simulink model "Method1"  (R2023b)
settings: Solver=FixedStepDiscrete  StartTime=0.0  StopTime=0.5  RelTol=1e-3
undefined symbols (not defined in the file): Datasheet, derived, set
libraries: fl_lib x14, nesl_utility x9, ee_lib x4, slpidlib x1, simulink x1, simulink_extras x1, spspowerguiLib x1

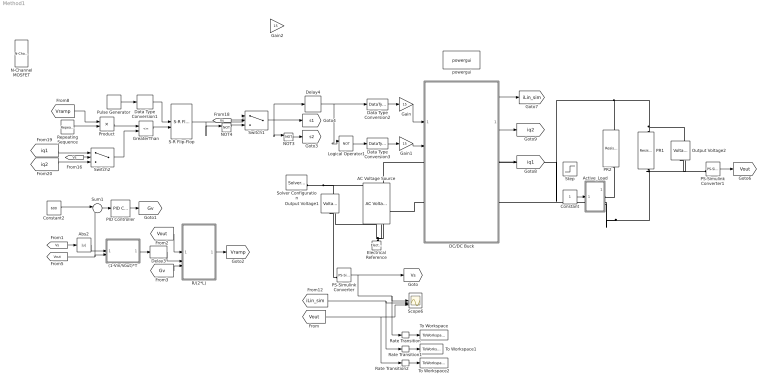
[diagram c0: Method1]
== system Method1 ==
  (1-Vin/Vout)*T : MATLAB Function  TreatAsAtomicUnit=on
  AC Voltage Source : fl_lib/Electrical/Electrical Sources/AC Voltage Source  amp=340 V  shift=0 deg  frequency=50 Hz  omega=0 rad/s
  Abs2 : Abs
  Active_Load : Subsystem
  Constant : Constant
  Constant2 : Constant  Value=600
  DC/DC Buck : Subsystem
  Data Type Conversion1 : DataTypeConversion
  Data Type Conversion2 : DataTypeConversion  OutDataTypeStr=double  RndMeth=Simplest
  Data Type Conversion3 : DataTypeConversion  OutDataTypeStr=double  RndMeth=Simplest
  Delay3 : Delay  DelayLength=10
  Delay4 : Delay  DelayLength=1
  Electrical Reference : fl_lib/Electrical/Electrical Elements/Electrical Reference
  Gain : Gain  Gain=15
  Gain1 : Gain  Gain=15
  Gain2 : Gain  Gain=15
  GreaterThan : RelationalOperator  Operator=<=  OutDataTypeStr=boolean  RndMeth=Simplest
  Logical Operator1 : Logic  Operator=NOT  AllPortsSameDT=off  OutDataTypeStr=boolean
  N-Channel MOSFET : ee_lib/Semiconductors & Converters/N-Channel MOSFET  paramTerminal=ee.enum.mosfet.numberOfTerminals.three  parameterization=ee.enum.mosfet.parameterization.datasheet  Beta=5.0 A/V^2  Rds=0.025 Ohm  Id=6.0 A  Vgs=10 V  Vth=1.7 V  Vth0=1.7 V  lam=0 1/V  gamma_vth=0.5 V^(1/2)  phib=0.5 V  Vth1=1.9071 V  Vbs1=-1 V  Vth2=2.066 V  Vbs2=-2 V  Tmeas=25 degC  Vgs_vec=[-1 0 0.74 1.41 2.02 2.57 3.06 3.51 3.91 4.27 4.6 4.9 5.17 5.41 5.63 5.82 6 6.16 6.31 6.44 6.56 6.67 6.81 6.97 7.16 7.37 7.61 7.89 8.21 8.57 8.98 9.45 9.99 10.61 11.31 12.11 13.03 14.08 15.28 16.65 18.21 20] V  Vds_vec=[0 0.1 1.1 2.1 3.1 4.1 5.1 6.1 7.1 8.1 9.1 10.1 11.1 12.1 13.1 14.1 15.1 16.1 17.1 18.1 19.1 20.1 30 40 50 60 70 80 90 100 110 120 130 140 150 160 170 180 190 200 210 220 230 240 250 260 270 280 290 300 310 320 330 340 350 360 370 380 390 400 410 420 430 440 450 460 470 480 490 500 510 520 530 540 550 560 570 580 590 600 610 620 630 640 650 660 670 680 690 700 710 720 730 740 750 760 770 780 790 8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  Vbs_vec=[0, -4, -6, -12] V  T_vec=[25;100;175] degC  Vth_vec=[.4, 1.2, 1.4, 1.45] V  Vth_mat=[.4, .35; 1.2, 1.15; 1.4, 1.35; 1.45, 1.4] V  Ids_mat=[0, 0, 0, 0, 0, 0, 0; 0, 0, 0, 0, 0, 0, 0; 0, .003, .0038, .0043, .0046, .0048, .0049; 0, .0055, .008, .009, .0095, .01, .0101; 0, .0115, .016, .018, .019, .0195, .02; 0, .0152, .0225, .0265, .028, .0295, .03] A  Ids_mat0=[0, 0, 0, 0, 0, 0, 0; 0, 0, 0, 0, 0, 0, 0; 0, .003, .0038, .0043, .0046, .0048, .0049; 0, .0055, .008, .009, .0095, .01, .0101; 0, .0115, .016, .018, .019, .0195, .02; 0, .0152, .0225, .0265, .028, .0295, .03] A  Ids_mat_3D=zeros(6, 7, 2) A  Ids_mat_3D0=zeros(6, 7, 2) A  IV_table_symmetry=ee.enum.mosfet.symmetricNIV.no  RS=0.0001 Ohm  RD=0.01 Ohm  RB=0.001 Ohm  C_param=ee.enum.mosfet.capacitanceParam.fixedciss  C_GS=270 pF  C_GD=80 pF  C_GB=0 pF  C_DS=0 pF  C_iss=350 pF  C_rss=80 pF  C_oss=0 pF  C_iss_vec=[720, 700, 590, 470, 390, 310] pF  C_rss_vec=[450, 400, 300, 190, 95, 55] pF  C_oss_vec=[900, 810, 690, 420, 270, 170] pF  C_GS_vec=[1.74124643236267e-09 1.74139785874173e-09 1.74141682364474e-09 1.74142233040577e-09 1.74142493418064e-09 1.7414278626316e-09 1.7414275761527e-09 1.7414298043219e-09 1.74143175237841e-09 1.74143352854757e-09 1.74143504370263e-09 1.74144584714017e-09 1.74145200961956e-09 1.74145583570439e-09 1.74145846494405e-09 1.74146041300056e-09 1.74146200454999e-09 1.7414633605501e-09 1.74146455102908e-09 1.74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  C_GD_vec=[9.31507143886424e-11 4.3042397570381e-11 3.61826985653635e-11 3.39318338671921e-11 3.26894767476145e-11 3.1388989876622e-11 3.01595816032143e-11 2.91496479963304e-11 2.82910007121519e-11 2.7539031803229e-11 2.68653098305279e-11 2.22551195235667e-11 1.9597372030282e-11 1.79177717186469e-11 1.67648978742733e-11 1.59040860828687e-11 1.52125260241458e-11 1.46254161714752e-11 1.41080543810653e-11 1.36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  C_GB_vec=[270, 300, 290, 280, 295, 255] pF  C_Vgs_vec=[-5 -3 -1 0 1 3 5 7 9 11 13 15 17 19] V  C_DS_vec=[1.23906948774915e-09;1.10548736992733e-09;1.00848198647898e-09;9.38035425004145e-10;8.74432653406217e-10;8.23194374689189e-10;5.9673868216423e-10;5.57776769053014e-10;5.31439700844806e-10;5.09747372298605e-10;4.9147030511283e-10;3.79228057666435e-10;3.19359971399718e-10;2.80602979827029e-10;2.54110264450675e-10;2.35046564409371e-10;2.20564585038808e-10;2.08974189970118e-10;1.9926781382197e-10;1.9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  C_Vds_vec=[0 1 2 3 4 5 6 7 8 9 10 20 30 40 50 60 70 80 90 100] V  V_GS_for_cap_data=0 V  charge_linearity_param=ee.enum.mosfet.cgdLinearity.constant  C_OX=200 pF  V_C_OX=-0.5 V  charge_linearity_param_vgb=ee.enum.mosfet.cgbLinearity.instantly  charge_linearity_param_with_vgb=ee.enum.mosfet.cgbLinearityWithSeparateCgb.instantly  Di_param=ee.enum.mosfet.diodeParam.no  IsDiode=1e-12 A  Vbi=0.6 V  n=1  Cj0Diode=0 pF  TT=50e-9 s  Tmeas_dio=25 degC  TableTypeNoT=ee.enum.mosfet.tableType.IfMat  TableType=ee.enum.diode.tableType.IfMat  IfVec=[.07, .12, .19, 1.75, 4.24, 7.32, 11.2] A  IfMat="[0 7.5e-06 0.1248618568 0.2497162136 0.3745705704 5.1758758156 13.872619052 25.668336366 40.124473959 56.940499125 75.890523695 96.795450744 119.50820242 143.90493397 169.87938371 197.33902678 226.20234059 256.39679287 287.85731962 320.52514703 354.34686179 389.27366528 425.26076668 462.26688303 500.25382274 539.18613541 579.03081476 619.75704463 661.33598032 703.74055915 746.94533536 790.9263354 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"  VfVecV=[.9, 1.15, 1.25, 1.5, 1.75, 2.17, 2.6, 2.85] V  VfMatV=[.9, 1.15, 1.25, 1.5, 1.75, 2.17, 2.6, 2.85; .58, .68, .75, 1.1, 1.38, 1.77, 2.27, 2.7] V  TjVec=[25 100 175] degC  VfVec=[0 0.75 1.5 2.25 3 3.75 4.5 5.25 6 6.75 7.5 8.25 9 9.75 10.5 11.25 12 12.75 13.5 14.25 15 15.75 16.5 17.25 18 18.75 19.5 20.25 21 21.75 22.5 23.25 24 24.75 25.5 26.25 27 27.75 28.5 29.25 30] V  IfVecV=[.1, .2, .5, 1, 2, 4, 7, 10] A  prmDatasheet=ee.enum.temperatureParameterization.none  prmEquCoeff=ee.enum.temperatureParameterization.none  dVth_dT=-6 mV/K  dVth0_dT=-6 mV/K  Rds_T2=0.037 Ohm  BEXDatasheet=-1.5  BEXEquCoeff=-1.5  etaisDatasheet=3  etaisEquCoeff=3  Tmeas2=125 degC  etaisTabulated=3  TdeviceDatasheet=25 degC  TdeviceEquCoeff=25 degC  TdeviceTabulated=25 degC  enable_faults=simscape.enum.onoff.off  fault_trigger=ee.enum.faults.faultTrigger.temporal  t_fault=inf s  max_permissible_Vgs=inf V  max_permissible_Vds=inf V  max_permissible_Vdb=inf V  max_permissible_Ids=inf A  t_fail_on_Ids=1 s  max_permissible_Idiode=inf A  t_fail_on_Idiode=1 s  max_permissible_dVdt=inf V/s  tau_fault=1e-3 s  fault_types=ee.enum.mosfet.faults.open  fault_types_4T=ee.enum.mosfet.faultsFourTerminals.open  RG_open=1e6 Ohm  RD_open=1000 Ohm  RS_open=1000 Ohm  RB_open=1000 Ohm  GDS_short=1000 1/Ohm  GDB_short=1000 1/Ohm  GSB_short=1000 1/Ohm  location_GOS=0  G_GOS=1000 1/Ohm  D_GOS=ee.enum.include.no  Is_GOS=0 A  Vbi_GOS=0.6 V  n_GOS=1  Cj0_GOS=0 pF  TT_GOS=50e-9 s  Beta_scale=100  dVth_faulted=0 V  lam_faulted=0 1/V  gamma_scale=100  dPhib_faulted=0 V  Vgs_vec_faulted=[-1, -.5, 2, 3, 4, 5] V  Vds_vec_faulted=[0, 2, 4, 8, 12, 16, 20] V  Vbs_vec_faulted=[0, -4, -6, -12] V  Vth_vec_faulted=[.4, 1.2, 1.4, 1.45] V  Vth_mat_faulted=[.4, .35; 1.2, 1.15; 1.4, 1.35; 1.45, 1.4] V  Ids_mat_faulted=[0, 0, 0, 0, 0, 0, 0; 0, 0, 0, 0, 0, 0, 0; 0, .003, .0038, .0043, .0046, .0048, .0049; 0, .0055, .008, .009, .0095, .01, .0101; 0, .0115, .016, .018, .019, .0195, .02; 0, .0152, .0225, .0265, .028, .0295, .03] A  Ids_mat0_faulted=[0, 0, 0, 0, 0, 0, 0; 0, 0, 0, 0, 0, 0, 0; 0, .003, .0038, .0043, .0046, .0048, .0049; 0, .0055, .008, .009, .0095, .01, .0101; 0, .0115, .016, .018, .019, .0195, .02; 0, .0152, .0225, .0265, .028, .0295, .03] A  Ids_mat_3D_faulted=zeros(6, 7, 2) A  Ids_mat_3D0_faulted=zeros(6, 7, 2) A  RS_faulted=0.0001 Ohm  RD_faulted=0.01 Ohm  RB_faulted=0.001 Ohm  IsDiode_faulted=0 A  Vbi_faulted=0.6 V  n_faulted=1  Cj0Diode_scale=100  TT_faulted=50e-9 s  IfVec_faulted=[.07, .12, .19, 1.75, 4.24, 7.32, 11.2] A  IfMat_faulted=[.07, .12, .19, 1.75, 4.24, 7.32, 11.2; .16, .3, .72, 2.14, 4.02, 6.35, 9.12] A  VfVecV_faulted=[.9, 1.15, 1.25, 1.5, 1.75, 2.17, 2.6, 2.85] V  VfMatV_faulted=[.9, 1.15, 1.25, 1.5, 1.75, 2.17, 2.6, 2.85; .58, .68, .75, 1.1, 1.38, 1.77, 2.27, 2.7] V  VfVec_faulted=[.5, .7, .9, 1.3, 1.7, 2.1, 2.5] V  IfVecV_faulted=[.1, .2, .5, 1, 2, 4, 7, 10] A  C_GS_scale=100  C_GD_scale=100  C_GB_scale=100  C_DS_scale=100  C_OX_scale=100  V_C_OX_faulted=-0.5 V  C_iss_vec_faulted=[720, 700, 590, 470, 390, 310] pF  C_rss_vec_faulted=[450, 400, 300, 190, 95, 55] pF  C_oss_vec_faulted=[900, 810, 690, 420, 270, 170] pF  C_GS_vec_faulted=[270, 300, 290, 280, 295, 255] pF  C_GD_vec_faulted=[450, 400, 300, 190, 95, 55] pF  C_GB_vec_faulted=[270, 300, 290, 280, 295, 255] pF  C_Vgs_vec_faulted=0 V  C_DS_vec_faulted=[450, 410, 390, 230, 175, 115] pF  C_Vds_vec_faulted=[.1, .3, 1, 3, 10, 30] V  V_GS_for_cap_data_faulted=0 V  i_g_specify=off  i_g_priority=None  i_g=0 A  i_g_nominal_specify=off  i_g_nominal_unit=A  i_g_nominal_value=1  i_d_specify=off  i_d_priority=None  i_d=0 A  i_d_nominal_specify=off  i_d_nominal_unit=A  i_d_nominal_value=1  i_b_specify=off  i_b_priority=None  i_b=0 A  i_b_nominal_specify=off  i_b_nominal_unit=A  i_b_nominal_value=1  voltage_gs_specify=off  voltage_gs_priority=None  voltage_gs=0 V  voltage_gs_nominal_specify=off  voltage_gs_nominal_unit=V  voltage_gs_nominal_value=1  voltage_ds_specify=off  voltage_ds_priority=None  voltage_ds=0 V  voltage_ds_nominal_specify=off  voltage_ds_nominal_unit=V  voltage_ds_nominal_value=1  voltage_bs_specify=off  voltage_bs_priority=None  voltage_bs=0 V  voltage_bs_nominal_specify=off  voltage_bs_nominal_unit=V  voltage_bs_nominal_value=1  v_Cgs_specify=off  v_Cgs_priority=High  v_Cgs=0 V  v_Cgs_nominal_specify=off  v_Cgs_nominal_unit=V  v_Cgs_nominal_value=1  v_Cds_specify=off  v_Cds_priority=High  v_Cds=0 V  v_Cds_nominal_specify=off  v_Cds_nominal_unit=V  v_Cds_nominal_value=1  v_Cbs_specify=off  v_Cbs_priority=High  v_Cbs=0 V  v_Cbs_nominal_specify=off  v_Cbs_nominal_unit=V  v_Cbs_nominal_value=1  faulted_specify=off  faulted_priority=None  faulted=0  faulted_nominal_specify=off  faulted_nominal_unit=1  faulted_nominal_value=1  thermal_network_parameterization=ee.enum.thermalNetworkTopology.junctionCase  Rth=[0, 10] K/W  Rth_Cauer=[1, 3, 10] K/W  Rth_Foster=[4, 6] K/W  thermal_mass_parameterization=ee.enum.thermalNetwork.timeconstant  thermal_mass=[0, 1] J/K  thermal_mass_Cauer=[.1, .3, 1] J/K  thermal_mass_Foster=[1.5, 3] J/K  thermal_time_constant=[0, 10] s  thermal_time_constant_Cauer=[1, 3, 10] s  thermal_time_constant_Foster=[6, 18] s  thermal_mass_initial_temperatures=[25, 25] degC  thermal_mass_initial_temperatures_Cauer=[25, 25, 25] degC  Tvec_initial_Foster=[25, 25, 25, 25] degC  max_permissible_temperature=inf K  t_fail_on_temperature=1 s  betaref=18 A/V^2  Vfbref=-1.1 V  gamma=3.5 V^(1/2)  phib2ref=1 V  thesatref=0.4 1/V  alpha=0  Vp=5e-2 V  thesrref=0 1/V  m=8  Tref=25 degC  Rsref=2e-3 Ohm  Rdref=0.17 Ohm  Rgref=8.4 Ohm  Rbref=2e-3 Ohm  Cox=1500 pF  Cgso=100 pF  Cgdo=14 pF  Isref=5.2e-13 A  Cj0=480 pF  Tprm=1  etabet=1.3  Stvfb=5e-4 V/K  Stphib=-8.5e-4 V/K  etasat=1.04  etasr=0.65  etar=0.95  etais=3  Tsim=25 degC  Ig_specify=off  Ig_priority=None  Ig=0 A  Ig_nominal_specify=off  Ig_nominal_unit=A  Ig_nominal_value=1  Ids_specify=off  Ids_priority=None  Ids=0 A  Ids_nominal_specify=off  Ids_nominal_unit=A  Ids_nominal_value=1  Ib_specify=off  Ib_priority=None  Ib=0 A  Ib_nominal_specify=off  Ib_nominal_unit=A  Ib_nominal_value=1  V_gs_specify=off  V_gs_priority=None  V_gs=0 V  V_gs_nominal_specify=off  V_gs_nominal_unit=V  V_gs_nominal_value=1  V_ds_specify=off  V_ds_priority=None  V_ds=0 V  V_ds_nominal_specify=off  V_ds_nominal_unit=V  V_ds_nominal_value=1  V_bs_specify=off  V_bs_priority=None  V_bs=0 V  V_bs_nominal_specify=off  V_bs_nominal_unit=V  V_bs_nominal_value=1  QGoverCox_specify=off  QGoverCox_priority=None  QGoverCox=0 V  QGoverCox_nominal_specify=off  QGoverCox_nominal_unit=V  QGoverCox_nominal_value=1  QDoverCox_specify=off  QDoverCox_priority=None  QDoverCox=0 V  QDoverCox_nominal_specify=off  QDoverCox_nominal_unit=V  QDoverCox_nominal_value=1  QBoverCox_specify=off  QBoverCox_priority=None  QBoverCox=0 V  QBoverCox_nominal_specify=off  QBoverCox_nominal_unit=V  QBoverCox_nominal_value=1  T0=[25, 25] degC  T0_Cauer=[25, 25, 25] degC
  NOT3 : Logic  Operator=NOT  IconShape=distinctive  AllPortsSameDT=off  OutDataTypeStr=boolean
  NOT4 : Logic  Operator=NOT  IconShape=distinctive  AllPortsSameDT=off  OutDataTypeStr=boolean
  Output Voltage1 : fl_lib/Electrical/Electrical Sensors/Voltage Sensor  Priority=0
  Output Voltage2 : fl_lib/Electrical/Electrical Sensors/Voltage Sensor  Priority=0
  PID Controller : slpidlib/PID Controller  Controller=PID  Form=Parallel  TimeDomain=Discrete-time  UseExternalTs=off  SampleTime=-1  IntegratorMethod=Forward Euler  FilterMethod=Forward Euler  ControllerParametersSource=internal  P=0  I=0.01  UseKiTs=off  D=0  N=100  UseFilter=on  TunerSelectOption=Transfer Function Based (PID Tuner App)  InitialConditionSource=internal  InitialConditionForIntegrator=0  InitialConditionForFilter=0  DifferentiatorICPrevScaledInput=0  ExternalReset=none  TrackingMode=off  Kt=1  LimitOutput=off  SatLimitsSource=internal  UpperSaturationLimit=0.9  LowerSaturationLimit=0  LinearizeAsGain=on  AntiWindupMode=none  Kb=1  LimitIntegrator=off  UpperIntegratorSaturationLimit=inf  LowerIntegratorSaturationLimit=-inf  POutMin=[]  POutMax=[]  IOutMin=[]  IOutMax=[]  DOutMin=[]  DOutMax=[]  NOutMin=[]  NOutMax=[]  SumOutMin=[]  SumOutMax=[]  SaturationOutMin=[]  SaturationOutMax=[]  PParamMin=[]  PParamMax=[]  IParamMin=[]  IParamMax=[]  DParamMin=[]  DParamMax=[]  NParamMin=[]  NParamMax=[]  KbParamMin=[]  KbParamMax=[]  KtParamMin=[]  KtParamMax=[]  KbOutMin=[]  KbOutMax=[]  KtOutMin=[]  KtOutMax=[]  IntegratorOutMin=[]  IntegratorOutMax=[]  FilterOutMin=[]  FilterOutMax=[]  SumI1OutMin=[]  SumI1OutMax=[]  SumI2OutMin=[]  SumI2OutMax=[]  SumI3OutMin=[]  SumI3OutMax=[]  SumI4OutMin=[]  SumI4OutMax=[]  SumDOutMin=[]  SumDOutMax=[]  DifferentiatorOutMin=[]  DifferentiatorOutMax=[]  FilterDiffOutCoefMin=[]  FilterDiffOutCoefMax=[]  ReciprocalOutMin=[]  ReciprocalOutMax=[]  SumDenOutMin=[]  SumDenOutMax=[]  SumNumOutMin=[]  SumNumOutMax=[]  DivideOutMin=[]  DivideOutMax=[]  UdiffTsProdOutMin=[]  UdiffTsProdOutMax=[]  NTsProdOutMin=[]  NTsProdOutMax=[]  UintegralTsProdOutMin=[]  UintegralTsProdOutMax=[]  UngainTsProdOutMin=[]  UngainTsProdOutMax=[]  ClampingZeroOutDataTypeStr=Inherit: Inherit via back propagation  ClampingZeroOutMin=[]  ClampingZeroOutMax=[]  FilterDenConstantOutDataTypeStr=Inherit: Inherit via back propagation  FilterDenConstantOutMin=[]  FilterDenConstantOutMax=[]  PCopyOutDataTypeStr=Inherit: Inherit via back propagation  PCopyOutMin=[]  PCopyOutMax=[]  NCopyOutDataTypeStr=Inherit: Inherit via back propagation  NCopyOutMin=[]  NCopyOutMax=[]  IntegratorContinuousStateAttributes=''  IntegratorStateMustResolveToSignalObject=off  IntegratorRTWStateStorageClass=Auto  FilterContinuousStateAttributes=''  FilterStateMustResolveToSignalObject=off  FilterRTWStateStorageClass=Auto  ParallelPVariant=InternalParameters  IdealPVariant=Disabled  IVariant=InternalParameters  DVariant=InternalParameters  IntegratorVariant=Discrete  SatVariant=Disabled  AWVariant=Passthrough  PCopyVariant=Disabled  TRVariant=Disabled  FdbkBlocksVariant=Forward  IdealPFdbkVariant=Disabled  SatFdbkVariant=Disabled  DerivativeFilterVariant=ForwardEulerFilter  NVariant=InternalParameters  NCopyVariant=Disabled  FilterICVariant=InternalICsFilter  IntegratorICVariant=InternalICs  ExternalResetVariant=Disabled  TRSumVariant=Passthrough  SumFdbkVariant=Disabled  SumVariant=Sum_PID  TsampFilterVariant=InternalTs  TsampNgainVariant=Passthrough  TsampIntegralVariant=Disabled_SignalSpec  ExternalSaturationOutDataTypeStr=Inherit: Same as second input
  PR1 : fl_lib/Electrical/Electrical Elements/Resistor  R=360 Ohm  i_specify=off  i_priority=None  i=0 A  i_nominal_specify=off  i_nominal_unit=A  i_nominal_value=1  v_specify=off  v_priority=None  v=0 V  v_nominal_specify=off  v_nominal_unit=V  v_nominal_value=1
  PR2 : fl_lib/Electrical/Electrical Elements/Resistor  R=360 Ohm  i_specify=off  i_priority=None  i=0 A  i_nominal_specify=off  i_nominal_unit=A  i_nominal_value=1  v_specify=off  v_priority=None  v=0 V  v_nominal_specify=off  v_nominal_unit=V  v_nominal_value=1
  PS-Simulink Converter : nesl_utility/PS-Simulink Converter  Priority=2  PhysicalDomain=network_engine_domain  SubClassName=ps_output  LeftPortType=input  RightPortType=output  PseudoPeriodic=off  Frequencies=[]  VectorFormat=1-D array  Unit=1  AffineConversion=off
  PS-Simulink Converter1 : nesl_utility/PS-Simulink Converter  Priority=2  PhysicalDomain=network_engine_domain  SubClassName=ps_output  LeftPortType=input  RightPortType=output  PseudoPeriodic=off  Frequencies=[]  VectorFormat=1-D array  Unit=1  AffineConversion=off
  Product : Product
  Pulse Generator : DiscretePulseGenerator  PulseType=Time based  Period=10e-6
  R/(2*L) : MATLAB Function  TreatAsAtomicUnit=on
  Rate Transition : RateTransition  OutPortSampleTime=1e-5
  Rate Transition1 : RateTransition  OutPortSampleTime=1e-5
  Rate Transition2 : RateTransition  OutPortSampleTime=1e-5
  Repeating Sequence : simulink/Sources/Repeating Sequence  rep_seq_t=[0 10e-6]  rep_seq_y=[1 0]
  S-R Flip-Flop : simulink_extras/Flip Flops/S-R Flip-Flop  initial_condition=0
  Scope6 : Scope  NumInputPorts=3
  Solver Configuration : nesl_utility/Solver Configuration  PhysicalDomain=network_engine_domain  SubClassName=solver  LeftPortType=input  RightPortType=generic  Tones=[]  Harmonics=[]  SimulateNoise=off  Profile=off  UseLocalSampling=off  EnableSwitchedLinearOptims=on  FrequencyDomain=off  UseCCode=off  RelTol=0.001  AbsTol=1e-06  MinStep=1e-09  ToWorkspace=off  RevertToSquareIcSolve=off  NumHomotopyIterations=100  PhasorMode=off  PhasorModeNumHarmonics=1  ConsistencySolver=NEWTON_FTOL  IndexReductionMethod=DerivativeReplacement  DoDC=off  ResidualTolerance=1e-08  ConsistencyTolSource=GLOBAL  ConsistencyAbsTol=0.001  ConsistencyRelTol=0.001  ConsistencyTolFactor=0.001  UseLocalSolver=on  LocalSolverChoice=NE_TRAPEZOIDAL_ADVANCER  ResolveIndetEquations=on  FunctionEvalNumThread=1  LocalSolverSampleTime=1e-7  DoFixedCost=on  MaxNonlinIter=3  MaxModeIter=2  ComputeImpulses=off  ImpulseIterations=2  LinearAlgebra=auto  LinearAlgebraNumThread=0  EquationFormulation=NE_TIME_EF  DelaysMemoryBudget=1024  AutomaticFiltering=on  FilteringTimeConstant=0.001  PartitionStorageMethod=AS_NEEDED  PartitionMemoryBudget=1024  PartitionMethod=ROBUST  MultibodyUseLocalSolver=off  MultibodyLocalSolverChoice=ODE1  MultibodyLocalSolverSampleTime=0.001
  Step : Step  Time=0.2  Before=1  After=0  SampleTime=0
  Sum1 : Sum  Inputs=|+-
  Switch1 : Switch  Criteria=u2 > Threshold
  Switch2 : Switch  Criteria=u2 > Threshold
  To Workspace : ToWorkspace  VariableName=Vs_method1  SaveFormat=Timeseries  SampleTime=-1
  To Workspace1 : ToWorkspace  VariableName=I_method1  SaveFormat=Timeseries  SampleTime=-1
  To Workspace2 : ToWorkspace  VariableName=Vout_method1  SaveFormat=Timeseries  SampleTime=-1
  powergui : spspowerguiLib/powergui  Priority=1  SimulationMode=Continuous  SampleTime=1e-6  frequency=60  Iterations=50  frequencyindice=60  Pbase=100e6  ErrMax=1e-4  UnitsV=kV  UnitsW=MW  buscounter=0  FunctionMessages=off  echomessages=off  EnableUseOfTLC=off  CurrentSourceSwitches=off  DisableSnubberDevices=off  DisableRonSwitches=off  DisableVfSwitches=off  DisplayEquations=off  AutomaticDiscreteSolvers=off  SolverType=Tustin/Backward Euler (TBE)  Interpol=off  ExternalGateDelay=off  methode=off  Ts=100  x0status=blocks  SPID=on  SwTol=0  HookPort=off  NonlinearTolerance=1e-4  nMaxIteration=100  ContinueOnMaxIteration=off  RestoreLinks=warning  ResistiveCurrentMeasurement=off  Frange=[0:2:500]  Ylog=off  Xlog=on  ShowGrid=off  save=off  variable=ZData  structure=0  ZoomFFT=off  StartTime=0.0  cycles=1  DisplayStyle=1  fundamental=60  FreqAxis=off  MaxFrequency=1000  frequencyindicesteady=1  RmsSteady=1  display=off
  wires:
  Logical Operator1/1 -> Data Type Conversion3/1
  Data Type Conversion2/1 -> Gain/1
  Data Type Conversion3/1 -> Gain1/1
  DC/DC Buck/1(I_sensor) -> [iLin_sim]
  Switch1/1 -> Delay4/1, NOT3/1, [s1]
  [Vout] -> Rate Transition2/1, Scope6/3
  [iLin_sim] -> Rate Transition1/1, Scope6/2
  S-R Flip-Flop/1 -> Switch1/1, NOT4/1
  NOT3/1 -> [s2]
  GreaterThan/1 -> S-R Flip-Flop/2
  NOT4/1 -> Switch1/3
  [Vs] -> Switch1/2
  Data Type Conversion1/1 -> S-R Flip-Flop/1
  Pulse Generator/1 -> Data Type Conversion1/1
  Repeating Sequence/1 -> Product/2
  Product/1 -> GreaterThan/1
  PS-Simulink Converter/1 -> [Vs], Rate Transition/1, Scope6/1
  (1-Vin/Vout)*T/1(Ton) -> Delay3/1
  [Gv] -> R/(2*L)/3(Gv)
  Delay3/1 -> R/(2*L)/2(Ton)
  R/(2*L)/1(y) -> [Vramp]
  PID Controller/1 -> [Gv]
  Sum1/1 -> PID Controller/1
  [Vs] -> Abs2/1
  [Vout] -> R/(2*L)/1(Vout)
  Constant2/1 -> Sum1/1
  [Vramp] -> Product/1
  [Vout] -> (1-Vin/Vout)*T/2(Vout), Sum1/2
  PS-Simulink Converter1/1 -> [Vout]
  Abs2/1 -> (1-Vin/Vout)*T/1(Vin)
  [Vs] -> Switch2/2
  [iq2] -> Switch2/3
  [iq1] -> Switch2/1
  Switch2/1 -> GreaterThan/2
  DC/DC Buck/3(iq1) -> [iq1]
  DC/DC Buck/2(iq2) -> [iq2]
  Delay4/1 -> Data Type Conversion2/1, Logical Operator1/1
  Rate Transition/1 -> To Workspace/1
  Rate Transition1/1 -> To Workspace1/1
  Rate Transition2/1 -> To Workspace2/1
  Gain/1 -> DC/DC Buck/1(In1)
  Gain1/1 -> DC/DC Buck/2(In2)
  Constant/1 -> Active_Load/1(In1)
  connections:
  PR1/RConn1 -- Output Voltage2/RConn2 -- Active_Load/RConn2 -- DC/DC Buck/RConn2
  Solver Configuration/RConn1 -- Output Voltage1/LConn1 -- AC Voltage Source/LConn1 -- DC/DC Buck/LConn1
  Electrical Reference/LConn1 -- DC/DC Buck/LConn2 -- Output Voltage1/RConn2 -- AC Voltage Source/RConn1
  PR1/LConn1 -- Output Voltage2/LConn1 -- DC/DC Buck/RConn1 -- PR2/LConn1
  PR2/RConn1 -- Active_Load/RConn1
  PS-Simulink Converter/LConn1 -- Output Voltage1/RConn1
  PS-Simulink Converter1/LConn1 -- Output Voltage2/RConn1

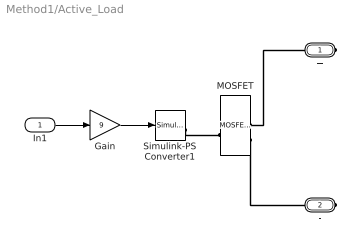
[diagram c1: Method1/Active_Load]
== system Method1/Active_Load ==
  In1 : Inport
  Gain : Gain  Gain=9
  MOSFET : ee_lib/Semiconductors & Converters/MOSFET (Ideal, Switching)  port_option=ee.enum.controlport.ps  Rds=0.2 Ohm  Goff=1e-6 1/Ohm  Vth=3 V  diode_param=ee.enum.converters.protectiondiode.nodynamics  diode_Vf=1.6 V  diode_Ron=0.001 Ohm  diode_Goff=1e-5 1/Ohm  diode_C=5e-8 F  diode_iRM=-235 A  diode_iF=300 A  diode_idot=-100 A/us  diode_trr_param=2  diode_trr_factor=3  diode_trr=70 ns  diode_Qrr=1.5e+3 s*uA  ids_specify=off  ids_priority=None  ids=0 A  ids_nominal_specify=off  ids_nominal_unit=A  ids_nominal_value=1  vds_specify=off  vds_priority=None  vds=0 V  vds_nominal_specify=off  vds_nominal_unit=V  vds_nominal_value=1  vgs_specify=off  vgs_priority=None  vgs=0 V  vgs_nominal_specify=off  vgs_nominal_unit=V  vgs_nominal_value=1  thermal_loss_option=ee.enum.converters.thermalLossOption.constantvalues  Von_data=[0, 1.8, 3.2, 6, 10, 16; 0, 2, 5.5, 9.5, 15, 25] V  Tj=[298.15, 448.15] K  Iout_data=[0, 20, 40, 60, 80, 100] A  Eon_data=[0, 55.04, 124.57, 235.53, 362.12; 0, 71.25, 161.25, 304.88, 468.75] * 1e-6 J  Eoff_data=[0, 18, 30, 56.1, 76.5; 0, 22.5, 37.5, 70.13, 95.63] * 1e-6 J  Eon_data_3D=[zeros(2, 5, 3)] J  Eoff_data_3D=[zeros(2, 5, 3)] J  Tj_loss=[298.15, 448.15] K  Iout_data_loss=[0, 10, 20, 30, 40] A  tabulateWithVds=false  Vds_loss=[0, 150, 300] V  Eon_scalar=22.86e-3 J  Eoff_scalar=17.14e-3 J  Voff=300 V  Iout_scalar=600 A  useCurrentFromPreviousCycle=false  useVoltageFromPreviousCycle=false  diodeModelType=ee.enum.converters.diodeModelType.pwl  diodeTableType=ee.enum.diode.tableType.IfMat  diode_IfMat=[.07, .12, .19, 1.75, 4.24, 7.32, 11.2; .16, .3, .72, 2.14, 4.02, 6.35, 9.12] A  diode_VfMat=[.9, 1.15, 1.25, 1.5, 1.75, 2.17, 2.6, 2.85; .58, .68, .75, 1.1, 1.38, 1.77, 2.27, 2.7] V  diode_TjVec=[25, 125] degC  diode_VfVec=[.5, .7, .9, 1.3, 1.7, 2.1, 2.5] V  diode_IfVec=[.1, .2, .5, 1, 2, 4, 7, 10] A  diode_Vr=-600 V  diode_Ls=150 nH  diode_Erec=0.03 J  diode_rec_loss_model=ee.enum.diode.reverseRecoveryModel.fixed  diode_ErecVal=0 J  diode_scaleWithIandV=true  diode_ErecMat=zeros(2, 3) J  diode_TjrecVec=[298.15, 398.15] K  diode_IfrecVec=[.1, 1, 10] A  diode_IrecVal=10 A  diode_VrecVal=10 V  diode_tFilter=1 / 1000 / 100 s  thermal_network_parameterization=ee.enum.thermalNetworkTopology.external  Rth=[.03, .2] K/W  Rth_Cauer=[.03, .1, .2] K/W  Rth_Foster=[.03, .2] K/W  thermal_mass_parameterization=ee.enum.thermalNetwork.timeconstant  thermal_mass=[3, 25] J/K  thermal_mass_Cauer=[3, 10, 25] J/K  thermal_mass_Foster=[33, 50] J/K  thermal_time_constant=[.1, 5] s  thermal_time_constant_Cauer=[.1, 1, 5] s  thermal_time_constant_Foster=[1, 10] s  thermal_mass_initial_temperatures=[25, 25] degC  thermal_mass_initial_temperatures_Cauer=[25, 25, 25] degC  junction_thermal_mass=0.1 J/K  Tvec_initial_Foster=[25, 25, 25, 25] degC  no_thermal_network=0  junction_temperature_specify=off  junction_temperature_priority=None  junction_temperature=25 degC  junction_temperature_nominal_specify=off  junction_temperature_nominal_unit=degC  junction_temperature_nominal_value=1  Qj_specify=off  Qj_priority=None  Qj=0 W  Qj_nominal_specify=off  Qj_nominal_unit=W  Qj_nominal_value=1  accumulatedSwitchingLosses_specify=off  accumulatedSwitchingLosses_priority=None  accumulatedSwitchingLosses=0 J
  Simulink-PS Converter1 : nesl_utility/Simulink-PS Converter  PhysicalDomain=network_engine_domain  SubClassName=ps_input  LeftPortType=input  RightPortType=output  PseudoPeriodic=off  Frequencies=[]  NoiseDistribution=none  NoiseParameters=[]  Unit=1  AffineConversion=off  FilteringAndDerivatives=provide  SimscapeFilterOrder=1  InputFilterTimeConstant=0.001  UdotUserProvided=0
  + : PMIOPort  Side=Right
  - : PMIOPort  Port=2  Side=Right
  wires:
  In1/1 -> Gain/1
  Gain/1 -> Simulink-PS Converter1/1
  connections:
  MOSFET/RConn2 -- -/RConn1
  MOSFET/RConn1 -- +/RConn1
  Simulink-PS Converter1/RConn1 -- MOSFET/LConn1

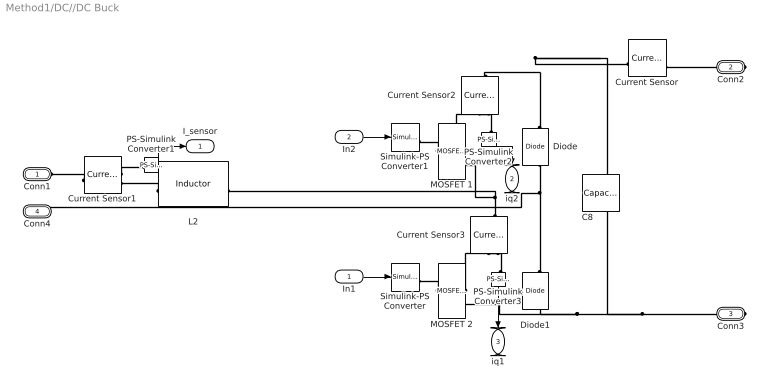
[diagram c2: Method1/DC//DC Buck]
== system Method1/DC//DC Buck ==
  In1 : Inport
  In2 : Inport  Port=2
  C8 : fl_lib/Electrical/Electrical Elements/Capacitor  c=0.1 mF  r=0.15 Ohm  g=0 1/Ohm  i_specify=off  i_priority=None  i=0 A  i_nominal_specify=off  i_nominal_unit=A  i_nominal_value=1  v_specify=off  v_priority=None  v=0 V  v_nominal_specify=off  v_nominal_unit=V  v_nominal_value=1  vc_specify=off  vc_priority=High  vc=0 V  vc_nominal_specify=off  vc_nominal_unit=V  vc_nominal_value=1
  Current Sensor{,1..3} (4 alike) : fl_lib/Electrical/Electrical Sensors/Current Sensor
  Diode : fl_lib/Electrical/Electrical Elements/Diode  Vf=0.6 V  Ron=0.3 Ohm  Goff=1e-8 1/Ohm  i_specify=off  i_priority=None  i=0 A  i_nominal_specify=off  i_nominal_unit=A  i_nominal_value=1  v_specify=off  v_priority=None  v=0 V  v_nominal_specify=off  v_nominal_unit=V  v_nominal_value=1
  Diode1 : fl_lib/Electrical/Electrical Elements/Diode  Vf=0.6 V  Ron=0.3 Ohm  Goff=1e-8 1/Ohm  i_specify=off  i_priority=None  i=0 A  i_nominal_specify=off  i_nominal_unit=A  i_nominal_value=1  v_specify=off  v_priority=None  v=0 V  v_nominal_specify=off  v_nominal_unit=V  v_nominal_value=1
  L2 : fl_lib/Electrical/Electrical Elements/Inductor  l=1 mH  r=0.0105 Ohm  g=0 1/Ohm  i_specify=off  i_priority=None  i=0 A  i_nominal_specify=off  i_nominal_unit=A  i_nominal_value=1  v_specify=off  v_priority=None  v=0 V  v_nominal_specify=off  v_nominal_unit=V  v_nominal_value=1  i_L_specify=off  i_L_priority=High  i_L=0 A  i_L_nominal_specify=off  i_L_nominal_unit=A  i_L_nominal_value=1
  MOSFET 1 : ee_lib/Semiconductors & Converters/MOSFET (Ideal, Switching)  Tag={'toolbox/physmod/elec/library/m/ee_lib_parts';'Semiconductors_and_Converters/MOSFET__Ideal__Switching_/Infineon/AIMW120R080M1.xml'}  port_option=ee.enum.controlport.ps  Rds=0.26 % Datasheet derived Ohm  Goff=2e-08 % Datasheet derived 1/Ohm  Vth=4.5 % Datasheet derived V  diode_param=ee.enum.converters.protectiondiode.nodynamics  diode_Vf=3.83 % Datasheet derived V  diode_Ron=0.048 % Datasheet derived Ohm  diode_Goff=1e-05 % Library default 1/Ohm  diode_C=50e-9 % Parameter not set F  diode_iRM=-235 % Parameter not set A  diode_iF=300 % Parameter not set A  diode_idot=-50 % Parameter not set A/us  diode_trr_param=ee.enum.converters.diodeReverseParam.trr_factor  diode_trr_factor=3 % Parameter not set  diode_trr=15 % Parameter not set us  diode_Qrr=1500 % Parameter not set s*uA  ids_specify=off  ids_priority=None  ids=0 A  ids_nominal_specify=off  ids_nominal_unit=A  ids_nominal_value=1  vds_specify=off  vds_priority=None  vds=0 V  vds_nominal_specify=off  vds_nominal_unit=V  vds_nominal_value=1  vgs_specify=off  vgs_priority=None  vgs=0 V  vgs_nominal_specify=off  vgs_nominal_unit=V  vgs_nominal_value=1  thermal_loss_option=ee.enum.converters.thermalLossOption.tabulated2d  Von_data=[0 0.21 0.42 0.63 0.84 1.22 1.66 2.09 2.57 3.09 3.61 4.18 4.91 5.65 6.38 7.33 8.31 9.43 10.71 12 13.81 15.69 17.78 19.87;0 0.41 0.81 1.22 1.63 2.03 2.59 3.16 3.72 4.29 4.99 5.68 6.4 7.26 8.12 8.98 10.07 11.23 12.38 13.89 15.4 17 18.83 20.65] % Datasheet derived V  Tj=[25 175] % Datasheet derived degC  Iout_data=[0 3.3 6.6 9.9 13.2 16.5 19.8 23.1 26.4 29.71 33.01 36.31 39.61 42.91 46.21 49.51 52.81 56.11 59.41 62.71 66.01 69.31 72.61 75.91] % Datasheet derived A  Eon_data=[0 2.39 17.04 31.69 46.33 60.98 75.63 90.28 104.92 119.57 134.22 148.87 163.51 178.16 192.81 207.46 222.1 236.75 251.37 265.31 279.25 293.19 307.13 321.07 335.01 348.95 362.89 376.83 390.77 405.86 424.27 442.67 461.07 479.48 497.88 517.66 543.15 568.63 594.12 619.6 645.09 670.57 696.06 721.54 747.83 777.14 806.45 835.76 865.07 894.38 923.69 953 982.31 1011.52 1040.61 1069.7 1098.79 1127.88 1156.96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  Eoff_data=[84.71 85.86 87.02 88.18 89.33 90.49 91.65 92.8 93.96 95.12 96.28 97.43 98.59 99.75 100.9 102.06 103.22 104.37 105.53 106.69 107.84 109 110.16 111.32 112.47 113.63 114.79 116.16 118 119.85 121.69 123.53 125.38 127.22 129.07 130.91 132.75 134.6 136.44 138.28 140.13 141.97 145.4 149.39 153.38 157.37 161.36 165.36 169.35 173.34 177.33 181.32 185.32 189.31 193.3 197.29 201.29 205.28 209.27 213.26 217.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  Eon_data_3D=[zeros(2, 5, 3)] % Parameter not set J  Eoff_data_3D=[zeros(2, 5, 3)] % Parameter not set J  Tj_loss=175 % Datasheet derived degC  Iout_data_loss=[0 0.55 1.11 1.66 2.22 2.77 3.33 3.88 4.43 4.99 5.54 6.1 6.65 7.2 7.76 8.31 8.87 9.42 9.98 10.53 11.08 11.64 12.19 12.75 13.3 13.86 14.41 14.96 15.52 16.07 16.63 17.18 17.74 18.29 18.84 19.4 19.95 20.51 21.06 21.61 22.17 22.72 23.28 23.83 24.39 24.94 25.49 26.05 26.6 27.16 27.71 28.27 28.82 29.37 29.93 30.48 31.04 31.59 32.15 32.7 33.25 33.81 34.36 34.92 35.47 36.02 36.58 37.13 37.69 38.24 38.8 39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  tabulateWithVds=false % Parameter not set  Vds_loss=[0, 150, 300] % Parameter not set V  Eon_scalar=22.86e-3 % Parameter not set J  Eoff_scalar=17.14e-3 % Parameter not set J  Voff=800 % Datasheet derived V  Iout_scalar=600 % Parameter not set A  useCurrentFromPreviousCycle=false  useVoltageFromPreviousCycle=false  diodeModelType=ee.enum.converters.diodeModelType.tabulated  diodeTableType=ee.enum.diode.tableType.IfMat  diode_IfMat=[0 0.102 0.2053 0.3102 3.8793 10.0341 16.4314 29.8;0 0.0638 0.4957 1.6585 6.589 12.4788 21.029 38.7605] % Datasheet derived A  diode_VfMat=[.9, 1.15, 1.25, 1.5, 1.75, 2.17, 2.6, 2.85; .58, .68, .75, 1.1, 1.38, 1.77, 2.27, 2.7] % Parameter not set V  diode_TjVec=[25 175] % Datasheet derived degC  diode_VfVec=[0 0.7 1.4 2.1 2.81 3.51 4.21 4.91] % Datasheet derived V  diode_IfVec=[.1, .2, .5, 1, 2, 4, 7, 10] % Parameter not set A  diode_Vr=-600 % Parameter not set V  diode_Ls=150 % Parameter not set nH  diode_Erec=0.03 % Parameter not set J  diode_rec_loss_model=ee.enum.diode.reverseRecoveryModel.fixed  diode_ErecVal=0 % Parameter not set J  diode_scaleWithIandV=false  diode_ErecMat=zeros(2, 3) % Parameter not set J  diode_TjrecVec=[298.15, 398.15] % Parameter not set K  diode_IfrecVec=[.1, 1, 10] % Parameter not set A  diode_IrecVal=10 % Parameter not set A  diode_VrecVal=10 % Parameter not set V  diode_tFilter=1 / 1000 / 100 % Parameter not set s  thermal_network_parameterization=ee.enum.thermalNetworkTopology.cauer  Rth=[.03, .2] % Parameter not set K/W  Rth_Cauer=[.03, .1, .2] % Parameter not set K/W  Rth_Foster=[.03, .2] % Parameter not set K/W  thermal_mass_parameterization=ee.enum.thermalNetwork.timeconstant  thermal_mass=[3, 25] % Parameter not set J/K  thermal_mass_Cauer=[3, 10, 25] % Parameter not set J/K  thermal_mass_Foster=[33, 50] % Parameter not set J/K  thermal_time_constant=[.1, 5] % Parameter not set s  thermal_time_constant_Cauer=[.1, 1, 5] % Parameter not set s  thermal_time_constant_Foster=[1, 10] % Parameter not set s  thermal_mass_initial_temperatures=[25, 25] % Parameter not set degC  thermal_mass_initial_temperatures_Cauer=[25, 25, 25] % Parameter not set degC  junction_thermal_mass=4.04 % Datasheet derived J/K  Tvec_initial_Foster=[25, 25, 25, 25] % Parameter not set degC  no_thermal_network=0 % Parameter not set  junction_temperature_specify=off  junction_temperature_priority=None  junction_temperature=25 degC  junction_temperature_nominal_specify=off  junction_temperature_nominal_unit=degC  junction_temperature_nominal_value=1  Qj_specify=off  Qj_priority=None  Qj=0 W  Qj_nominal_specify=off  Qj_nominal_unit=W  Qj_nominal_value=1  accumulatedSwitchingLosses_specify=off  accumulatedSwitchingLosses_priority=None  accumulatedSwitchingLosses=0 J
  MOSFET 2 : ee_lib/Semiconductors & Converters/MOSFET (Ideal, Switching)  Tag={'toolbox/physmod/elec/library/m/ee_lib_parts';'Semiconductors_and_Converters/MOSFET__Ideal__Switching_/Infineon/AIMW120R080M1.xml'}  port_option=ee.enum.controlport.ps  Rds=0.26 % Datasheet derived Ohm  Goff=2e-08 % Datasheet derived 1/Ohm  Vth=4.5 % Datasheet derived V  diode_param=ee.enum.converters.protectiondiode.nodynamics  diode_Vf=3.83 % Datasheet derived V  diode_Ron=0.048 % Datasheet derived Ohm  diode_Goff=1e-05 % Library default 1/Ohm  diode_C=50e-9 % Parameter not set F  diode_iRM=-235 % Parameter not set A  diode_iF=300 % Parameter not set A  diode_idot=-50 % Parameter not set A/us  diode_trr_param=ee.enum.converters.diodeReverseParam.trr_factor  diode_trr_factor=3 % Parameter not set  diode_trr=15 % Parameter not set us  diode_Qrr=1500 % Parameter not set s*uA  ids_specify=off  ids_priority=None  ids=0 A  ids_nominal_specify=off  ids_nominal_unit=A  ids_nominal_value=1  vds_specify=off  vds_priority=None  vds=0 V  vds_nominal_specify=off  vds_nominal_unit=V  vds_nominal_value=1  vgs_specify=off  vgs_priority=None  vgs=0 V  vgs_nominal_specify=off  vgs_nominal_unit=V  vgs_nominal_value=1  thermal_loss_option=ee.enum.converters.thermalLossOption.tabulated2d  Von_data=[0 0.21 0.42 0.63 0.84 1.22 1.66 2.09 2.57 3.09 3.61 4.18 4.91 5.65 6.38 7.33 8.31 9.43 10.71 12 13.81 15.69 17.78 19.87;0 0.41 0.81 1.22 1.63 2.03 2.59 3.16 3.72 4.29 4.99 5.68 6.4 7.26 8.12 8.98 10.07 11.23 12.38 13.89 15.4 17 18.83 20.65] % Datasheet derived V  Tj=[25 175] % Datasheet derived degC  Iout_data=[0 3.3 6.6 9.9 13.2 16.5 19.8 23.1 26.4 29.71 33.01 36.31 39.61 42.91 46.21 49.51 52.81 56.11 59.41 62.71 66.01 69.31 72.61 75.91] % Datasheet derived A  Eon_data=[0 2.39 17.04 31.69 46.33 60.98 75.63 90.28 104.92 119.57 134.22 148.87 163.51 178.16 192.81 207.46 222.1 236.75 251.37 265.31 279.25 293.19 307.13 321.07 335.01 348.95 362.89 376.83 390.77 405.86 424.27 442.67 461.07 479.48 497.88 517.66 543.15 568.63 594.12 619.6 645.09 670.57 696.06 721.54 747.83 777.14 806.45 835.76 865.07 894.38 923.69 953 982.31 1011.52 1040.61 1069.7 1098.79 1127.88 1156.96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  Eoff_data=[84.71 85.86 87.02 88.18 89.33 90.49 91.65 92.8 93.96 95.12 96.28 97.43 98.59 99.75 100.9 102.06 103.22 104.37 105.53 106.69 107.84 109 110.16 111.32 112.47 113.63 114.79 116.16 118 119.85 121.69 123.53 125.38 127.22 129.07 130.91 132.75 134.6 136.44 138.28 140.13 141.97 145.4 149.39 153.38 157.37 161.36 165.36 169.35 173.34 177.33 181.32 185.32 189.31 193.3 197.29 201.29 205.28 209.27 213.26 217.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  Eon_data_3D=[zeros(2, 5, 3)] % Parameter not set J  Eoff_data_3D=[zeros(2, 5, 3)] % Parameter not set J  Tj_loss=175 % Datasheet derived degC  Iout_data_loss=[0 0.55 1.11 1.66 2.22 2.77 3.33 3.88 4.43 4.99 5.54 6.1 6.65 7.2 7.76 8.31 8.87 9.42 9.98 10.53 11.08 11.64 12.19 12.75 13.3 13.86 14.41 14.96 15.52 16.07 16.63 17.18 17.74 18.29 18.84 19.4 19.95 20.51 21.06 21.61 22.17 22.72 23.28 23.83 24.39 24.94 25.49 26.05 26.6 27.16 27.71 28.27 28.82 29.37 29.93 30.48 31.04 31.59 32.15 32.7 33.25 33.81 34.36 34.92 35.47 36.02 36.58 37.13 37.69 38.24 38.8 39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  tabulateWithVds=false % Parameter not set  Vds_loss=[0, 150, 300] % Parameter not set V  Eon_scalar=22.86e-3 % Parameter not set J  Eoff_scalar=17.14e-3 % Parameter not set J  Voff=800 % Datasheet derived V  Iout_scalar=600 % Parameter not set A  useCurrentFromPreviousCycle=false  useVoltageFromPreviousCycle=false  diodeModelType=ee.enum.converters.diodeModelType.tabulated  diodeTableType=ee.enum.diode.tableType.IfMat  diode_IfMat=[0 0.102 0.2053 0.3102 3.8793 10.0341 16.4314 29.8;0 0.0638 0.4957 1.6585 6.589 12.4788 21.029 38.7605] % Datasheet derived A  diode_VfMat=[.9, 1.15, 1.25, 1.5, 1.75, 2.17, 2.6, 2.85; .58, .68, .75, 1.1, 1.38, 1.77, 2.27, 2.7] % Parameter not set V  diode_TjVec=[25 175] % Datasheet derived degC  diode_VfVec=[0 0.7 1.4 2.1 2.81 3.51 4.21 4.91] % Datasheet derived V  diode_IfVec=[.1, .2, .5, 1, 2, 4, 7, 10] % Parameter not set A  diode_Vr=-600 % Parameter not set V  diode_Ls=150 % Parameter not set nH  diode_Erec=0.03 % Parameter not set J  diode_rec_loss_model=ee.enum.diode.reverseRecoveryModel.fixed  diode_ErecVal=0 % Parameter not set J  diode_scaleWithIandV=false  diode_ErecMat=zeros(2, 3) % Parameter not set J  diode_TjrecVec=[298.15, 398.15] % Parameter not set K  diode_IfrecVec=[.1, 1, 10] % Parameter not set A  diode_IrecVal=10 % Parameter not set A  diode_VrecVal=10 % Parameter not set V  diode_tFilter=1 / 1000 / 100 % Parameter not set s  thermal_network_parameterization=ee.enum.thermalNetworkTopology.cauer  Rth=[.03, .2] % Parameter not set K/W  Rth_Cauer=[.03, .1, .2] % Parameter not set K/W  Rth_Foster=[.03, .2] % Parameter not set K/W  thermal_mass_parameterization=ee.enum.thermalNetwork.timeconstant  thermal_mass=[3, 25] % Parameter not set J/K  thermal_mass_Cauer=[3, 10, 25] % Parameter not set J/K  thermal_mass_Foster=[33, 50] % Parameter not set J/K  thermal_time_constant=[.1, 5] % Parameter not set s  thermal_time_constant_Cauer=[.1, 1, 5] % Parameter not set s  thermal_time_constant_Foster=[1, 10] % Parameter not set s  thermal_mass_initial_temperatures=[25, 25] % Parameter not set degC  thermal_mass_initial_temperatures_Cauer=[25, 25, 25] % Parameter not set degC  junction_thermal_mass=4.04 % Datasheet derived J/K  Tvec_initial_Foster=[25, 25, 25, 25] % Parameter not set degC  no_thermal_network=0 % Parameter not set  junction_temperature_specify=off  junction_temperature_priority=None  junction_temperature=25 degC  junction_temperature_nominal_specify=off  junction_temperature_nominal_unit=degC  junction_temperature_nominal_value=1  Qj_specify=off  Qj_priority=None  Qj=0 W  Qj_nominal_specify=off  Qj_nominal_unit=W  Qj_nominal_value=1  accumulatedSwitchingLosses_specify=off  accumulatedSwitchingLosses_priority=None  accumulatedSwitchingLosses=0 J
  PS-Simulink Converter1 : nesl_utility/PS-Simulink Converter  PhysicalDomain=network_engine_domain  SubClassName=ps_output  LeftPortType=input  RightPortType=output  PseudoPeriodic=off  Frequencies=[]  VectorFormat=inherit  Unit=inherit  AffineConversion=off
  PS-Simulink Converter2 : nesl_utility/PS-Simulink Converter  PhysicalDomain=network_engine_domain  SubClassName=ps_output  LeftPortType=input  RightPortType=output  PseudoPeriodic=off  Frequencies=[]  VectorFormat=inherit  Unit=inherit  AffineConversion=off
  PS-Simulink Converter3 : nesl_utility/PS-Simulink Converter  PhysicalDomain=network_engine_domain  SubClassName=ps_output  LeftPortType=input  RightPortType=output  PseudoPeriodic=off  Frequencies=[]  VectorFormat=inherit  Unit=inherit  AffineConversion=off
  Simulink-PS Converter : nesl_utility/Simulink-PS Converter  PhysicalDomain=network_engine_domain  SubClassName=ps_input  LeftPortType=input  RightPortType=output  PseudoPeriodic=off  Frequencies=[]  NoiseDistribution=none  NoiseParameters=[]  Unit=1  AffineConversion=off  FilteringAndDerivatives=provide  SimscapeFilterOrder=1  InputFilterTimeConstant=0.001  UdotUserProvided=0
  Simulink-PS Converter1 : nesl_utility/Simulink-PS Converter  PhysicalDomain=network_engine_domain  SubClassName=ps_input  LeftPortType=input  RightPortType=output  PseudoPeriodic=off  Frequencies=[]  NoiseDistribution=none  NoiseParameters=[]  Unit=1  AffineConversion=off  FilteringAndDerivatives=provide  SimscapeFilterOrder=1  InputFilterTimeConstant=0.001  UdotUserProvided=0
  Conn1 : PMIOPort  Side=Left
  Conn2 : PMIOPort  Port=2  Side=Right
  Conn3 : PMIOPort  Port=3  Side=Right
  Conn4 : PMIOPort  Port=4  Side=Left
  I_sensor : Outport  VectorParamsAs1DForOutWhenUnconnected=off
  iq2 : Outport  Port=2  VectorParamsAs1DForOutWhenUnconnected=off
  iq1 : Outport  Port=3  VectorParamsAs1DForOutWhenUnconnected=off
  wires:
  In2/1 -> Simulink-PS Converter1/1
  In1/1 -> Simulink-PS Converter/1
  PS-Simulink Converter1/1 -> I_sensor/1
  PS-Simulink Converter3/1 -> iq1/1
  PS-Simulink Converter2/1 -> iq2/1
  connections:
  Conn3/RConn1 -- C8/RConn1 -- MOSFET 2/RConn2 -- Diode1/LConn1
  Current Sensor3/LConn1 -- MOSFET 1/RConn2 -- L2/RConn1
  L2/LConn1 -- Current Sensor1/RConn2
  Diode/LConn1 -- Conn4/RConn1 -- Diode1/RConn1
  Diode/RConn1 -- Current Sensor2/LConn1 -- C8/LConn1 -- Current Sensor/LConn1
  Current Sensor1/LConn1 -- Conn1/RConn1
  Current Sensor1/RConn1 -- PS-Simulink Converter1/LConn1
  Current Sensor/RConn2 -- Conn2/RConn1
  MOSFET 1/RConn1 -- Current Sensor2/RConn2
  MOSFET 2/RConn1 -- Current Sensor3/RConn2
  PS-Simulink Converter2/LConn1 -- Current Sensor2/RConn1
  PS-Simulink Converter3/LConn1 -- Current Sensor3/RConn1
  MOSFET 1/LConn1 -- Simulink-PS Converter1/RConn1
  MOSFET 2/LConn1 -- Simulink-PS Converter/RConn1

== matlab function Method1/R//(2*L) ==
function y = fcn(Vout, Ton, Gv)

% current-sense resistor for the current transformer. 
%Here, Rsense here in the simulation is Ron of the MOSFET. Thus, Rsense = 0.01;
Rsense = 1;
L = 1e-3;

y = (Gv + Ton/(2*L)*Rsense)*Vout;

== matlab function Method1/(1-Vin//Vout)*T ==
function Ton = fcn(Vin, Vout)

T = 10e-6; 

Ton = ((Vout-Vin)/Vout)*T;
